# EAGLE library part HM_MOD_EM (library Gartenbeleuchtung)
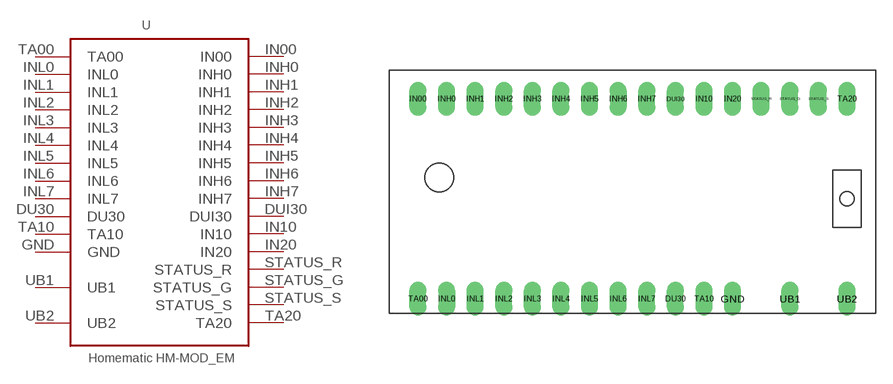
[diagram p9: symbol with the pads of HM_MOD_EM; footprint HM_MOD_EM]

Designator prefix -

## HM_MOD_EM  [HM_MOD_EM]
DU30  DU30
DUI30  DUI30
GND  GND  pwr
IN00  IN00
IN10  IN10
IN20  IN20
INH0  INH0
INH1  INH1
INH2  INH2
INH3  INH3
INH4  INH4
INH5  INH5
INH6  INH6
INH7  INH7
INL0  INL0
INL1  INL1
INL2  INL2
INL3  INL3
INL4  INL4
INL5  INL5
INL6  INL6
INL7  INL7
STATUS_G  STATUS_G
STATUS_R  STATUS_R
STATUS_S  STATUS_S
TA00  TA00
TA10  TA10
TA20  TA20
UB1  UB1  pwr
UB2  UB2  pwr

## Footprint HM_MOD_EM (pad centres in mm)
drill 1 pad 1.422 long: DU30 22.86,0; DUI30 22.86,17.78; GND 27.94,0; IN00 0,17.78; IN10 25.4,17.78; IN20 27.94,17.78; INH0 2.54,17.78; INH1 5.08,17.78; INH2 7.62,17.78; INH3 10.16,17.78; INH4 12.7,17.78; INH5 15.24,17.78; INH6 17.78,17.78; INH7 20.32,17.78; INL0 2.54,0; INL1 5.08,0; INL2 7.62,0; INL3 10.16,0; INL4 12.7,0; INL5 15.24,0; INL6 17.78,0; INL7 20.32,0; STATUS_G 33.02,17.78; STATUS_R 30.48,17.78; STATUS_S 35.56,17.78; TA00 0,0; TA10 25.4,0; TA20 38.1,17.78; UB1 33.02,0; UB2 38.1,0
